(* Logix 5000 AddOnInstructionDefinition export Bronkhorst_Basic_REAL_Input; software revision 37.00 *)

ADD_ON_INSTRUCTION Bronkhorst_Basic_REAL_Input   (* revision 1.0, vendor Bronkhorst High-Tech B.V. *)
// Extract data from the Basic REAL input connection (in to controller from device)
VAR_IN_OUT
   DataIn : SINT[5]; {required}
END_VAR
VAR_OUTPUT
   Status : SINT; {visible}
   Measure : REAL; {visible}
END_VAR

ROUTINE Logic   (* structured text *)
   Status := DataIn[0];
   COP(DataIn[1], Measure, 1);
END_ROUTINE
END_ADD_ON_INSTRUCTION

ADD_ON_INSTRUCTION Bronkhorst_Basic_REAL_Output   (* revision 1.0, vendor Bronkhorst High-Tech B.V. *)
// Fill data for the Basic REAL output connection (out from controller to device)
VAR_IN_OUT
   DataOut : SINT[4]; {required}
END_VAR
VAR_INPUT
   Setpoint : REAL; {visible}
END_VAR

ROUTINE Logic   (* structured text *)
   COP(Setpoint, DataOut[0], 4);
END_ROUTINE
END_ADD_ON_INSTRUCTION
